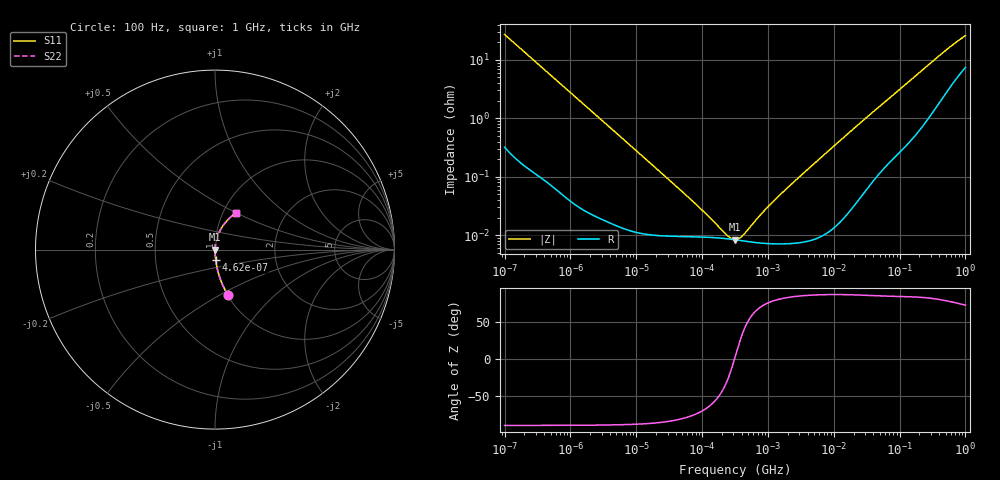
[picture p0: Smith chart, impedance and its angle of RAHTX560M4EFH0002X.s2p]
! RAHTX560M4EFH0002X  S-PARAMETER MODEL  (AEC-Q200 qualified)
! Model Generated by ELNA Corporation (http://www.ty-top.com)
! Version 1.0
! ELNA Control No. 231122
! Copyright (c) 2023 ELNA CO.,LTD. All Rights Reserved.
! Products Name : CONDUCTIVE POLYMER HYBRID ALUMINUM ELECTROLYTIC CAPACITORS
! Characteristics :
!  Capacitance  :  56uF  ,  Rated voltage  :  63V
!  Operating Temp. Range  :  -55 to +135 degC  ,  Endurance  :  4000hr at 135 degC
!  Dimension D  :  10mm  ,  Dimension L  :  10mm
! Frequency Range : 100Hz - 1GHz
! External Node Assignments :
!  1  o---| |---o  2
# MHz S RI R 50
!Freq[MHz].  S11 Real  S11 Imag  S21 Real  S21 Imag  S12 Real  S12 Imag  S22 Real  S22 Imag
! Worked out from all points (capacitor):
!   401 points, 100 Hz to 1 GHz, reference 50 ohm
!   read as one part in series: C = 58.5 uF near 108 Hz
!   lowest |Z| = 8.39 mohm at 316.2 kHz (marker M1)
!   series resonance near 309.6 kHz, so ESL is about 4.5 nH
!   S11 on the Smith chart (normalised r, x): 100 Hz: 1.01, -0.54; 462 Hz: 1.00, -0.12; 1 GHz: 1.15, +0.50
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0.0001  0.0716 -0.2519  0.9284 0.2519  0.9284 0.2519  0.0716 -0.2519
0.000113  0.0573 -0.2268  0.9427 0.2268  0.9427 0.2268  0.0573 -0.2268
0.000198  0.02 -0.1345  0.98 0.1345  0.98 0.1345  0.02 -0.1345
0.000462  0.00427 -0.059  0.9957 0.059  0.9957 0.059  0.00427 -0.059
0.001488  0.000625 -0.0186  0.9994 0.0186  0.9994 0.0186  0.000625 -0.0186
0.022131  0.0001 -0.00126  0.9999 0.00126  0.9999 0.00126  0.0001 -0.00126
0.090678  9.37e-05 -0.000285  0.9999 0.000285  0.9999 0.000285  9.37e-05 -0.000285
0.220039  8.81e-05 -6.54e-05  0.9999 6.54e-05  0.9999 6.54e-05  8.81e-05 -6.54e-05
0.248313  8.68e-05 -4.21e-05  0.9999 4.21e-05  0.9999 4.21e-05  8.68e-05 -4.21e-05
0.316228  8.38e-05 4.09e-06  0.9999 -4.09e-06  0.9999 -4.09e-06  8.38e-05 4.09e-06
0.386812  8.12e-05 4.37e-05  0.9999 -4.37e-05  0.9999 -4.37e-05  8.12e-05 4.37e-05
0.436516  7.96e-05 6.88e-05  0.9999 -6.88e-05  0.9999 -6.88e-05  7.96e-05 6.88e-05
0.767361  7.37e-05 0.00021  0.9999 -0.00021  0.9999 -0.00021  7.37e-05 0.00021
1.148154  7.17e-05 0.000353  0.9999 -0.000353  0.9999 -0.000353  7.17e-05 0.000353
2.018366  7.21e-05 0.000658  0.9999 -0.000658  0.9999 -0.000658  7.21e-05 0.000658
4.704354  8.53e-05 0.00157  0.9999 -0.00157  0.9999 -0.00157  8.53e-05 0.00157
21.75204  0.000403 0.0072  0.9996 -0.0072  0.9996 -0.0072  0.000403 0.0072
69.9842  0.00223 0.022  0.9978 -0.022  0.9978 -0.022  0.00223 0.022
184.0772  0.00854 0.055  0.9915 -0.055  0.9915 -0.055  0.00854 0.055
429.0422  0.0344 0.1175  0.9656 -0.1175  0.9656 -0.1175  0.0344 0.1175
695.825  0.073 0.1676  0.927 -0.1676  0.927 -0.1676  0.073 0.1676
1000  0.1166 0.2053  0.8834 -0.2053  0.8834 -0.2053  0.1166 0.2053
